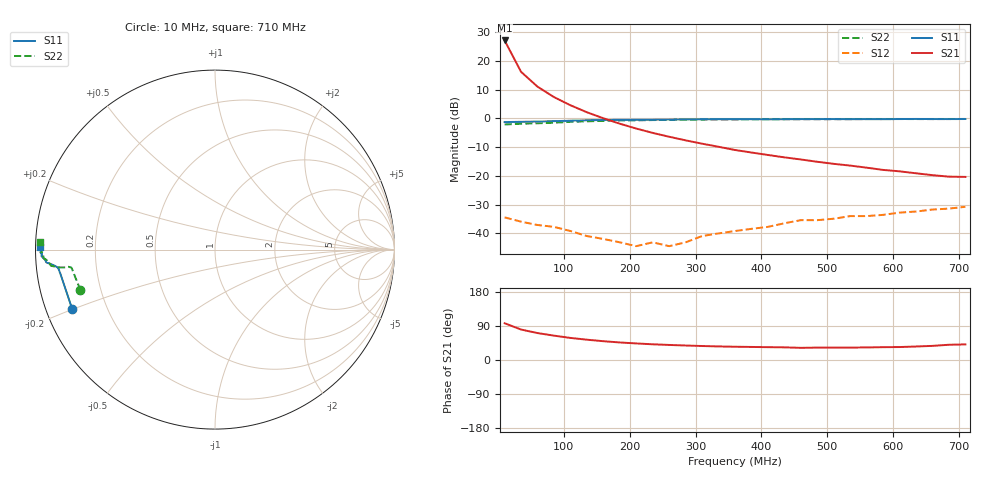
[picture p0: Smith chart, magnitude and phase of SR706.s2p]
!  POLYFET RF DEVICES
!  S PARAMETERS FOR
!  SR706 (EACH SIDE)
!  VDS=28, IDQ=600MA
! Date: Thu Mar 30 10:48:53 2000
# MHZ S MA R 50
!FREQ-MHZ MAG[S11] ANG[S11] MAG[S21] ANG[S21] MAG[S12] ANG[S12] MAG[S22] ANG[S22]
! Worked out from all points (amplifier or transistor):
!   29 points, 10 MHz to 710 MHz, reference 50 ohm
!   highest |S21| = 27.1 dB at 10 MHz (marker M1)
!   |S21| within 3 dB of that: start of sweep to 16.88 MHz
!   unconditionally stable (mu >= 1): 192.6 MHz to end of sweep
!   at 110 MHz: K = 0.47, MSG = 21.9 dB, |S12| = -39.2 dB
!   at 360 MHz: K = 1.18, MAG = 11.5 dB, |S12| = -39.2 dB
!   at 710 MHz: K = 1.21, MAG = 2.4 dB, |S12| = -30.8 dB
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10  0.862 -157.2  22.62 97.0  0.019 5.4  0.783 -163.2
35  0.872 -171.2  6.444 80.4  0.016 -3.1  0.806 -172.9
60  0.88 -173.3  3.556 71.1  0.014 -11.8  0.822 -173.3
85  0.894 -174.1  2.345 64.3  0.013 -13.1  0.839 -173.2
110  0.912 -174.7  1.69 58.3  0.011 -10.6  0.87 -173.4
135  0.926 -175.2  1.277 53.6  0.009 -6.6  0.888 -173.7
160  0.938 -175.5  1.004 49.6  0.008 1.9  0.905 -174.1
185  0.943 -175.7  0.808 46.3  0.007 -1.3  0.918 -174.4
210  0.945 -176.1  0.665 43.7  0.006 23.2  0.924 -175.1
235  0.948 -176.5  0.559 41.4  0.007 36.7  0.934 -175.8
260  0.954 -177.0  0.479 39.7  0.006 52.1  0.939 -176.4
285  0.959 -177.3  0.415 38.2  0.007 65.3  0.948 -176.9
310  0.965 -177.7  0.363 36.9  0.009 68.2  0.955 -177.1
360  0.966 -178.1  0.282 35.0  0.011 76.7  0.958 -178.5
410  0.964 -178.6  0.231 33.9  0.013 86.8  0.963 -179.0
460  0.971 -178.9  0.193 32.1  0.017 87.3  0.966 -179.1
485  0.971 -179.1  0.176 32.7  0.017 89.6  0.968 -179.8
535  0.968 -179.4  0.151 32.7  0.02 91.2  0.97 179.4
560  0.97 -179.7  0.139 33.2  0.02 95.3  0.971 179.0
610  0.973 179.9  0.12 34.2  0.023 99.2  0.974 178.8
685  0.971 179.9  0.097 40.2  0.027 102.4  0.975 177.9
710  0.974 179.3  0.096 41.2  0.029 102.3  0.977 177.7
